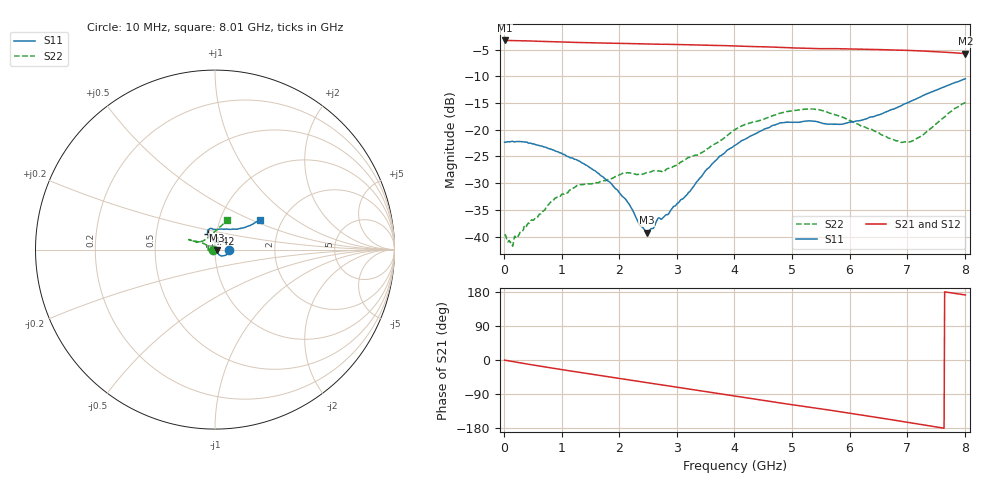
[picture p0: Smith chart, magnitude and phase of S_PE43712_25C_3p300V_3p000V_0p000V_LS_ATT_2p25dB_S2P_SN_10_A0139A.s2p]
! DEVICE ID: PE43712
! File Path: z:\PE43713\PE43713_CHAR_NOM_04292014\AMB\3p300\LS_ATT_2p25dB\PE43713_AMB_3p300V_3p000V_0p000V_LS_ATT_2p25dB_S2P_SN_10_A0139A.s2p
! Serial: 10
! Lot: A0139A
! Temp: 25C
! VDD: 3.300
! VSS: 0.000
! Control_Hi: 3.000
! Control_Lo: 0.000
! Attenuation Step: 2.25dB
! Port 1: RF1
! Port 2: RF2
! ThroughPath:1-2
! IDD: 0.0001467323
! ISS: -1.32e-007
#  Hz  S  RI  R  50
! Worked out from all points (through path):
!   801 points, 10 MHz to 8.01 GHz, reference 50 ohm
!   highest |S21| = -3.29 dB at 10 MHz (marker M1); lowest = -5.7 dB at 8.01 GHz (marker M2)
!   group delay of S21, straight-line fit = 64.5 ps
!   lowest |S11| = -39.3 dB at 2.48 GHz (marker M3), VSWR 1.02, Z = 51.1 - j0.227 ohm
!   |S11| at or under -10 dB: start of sweep to end of sweep
!   |S22| runs from -41.8 to -14.9 dB; largest |S21 - S12| = 0.002
!   S11 on the Smith chart (normalised r, x): 10 MHz: 1.17, -0.00; 4.42 GHz: 0.91, +0.16; 8.01 GHz: 1.55, +0.56
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1e7  0.0765 -0.000436  0.685 -0.00397  0.6847 -0.00374  -0.0103 -0.000149
1.3e8  0.0777 -0.00596  0.6821 -0.0422  0.682 -0.0421  -0.00858 -0.00171
9e8  0.0534 -0.0332  0.6128 -0.2592  0.6127 -0.259  -0.0179 -0.0144
1.35e9  0.0346 -0.0348  0.546 -0.3613  0.5458 -0.3612  -0.0268 -0.015
1.86e9  0.0196 -0.0246  0.4541 -0.4587  0.4541 -0.4586  -0.0342 -0.00646
2.14e9  0.0122 -0.0173  0.3965 -0.504  0.3965 -0.5037  -0.0396 -0.00107
2.35e9  0.0103 -0.00777  0.3501 -0.5332  0.3501 -0.5331  -0.0381 0.00486
2.48e9  0.0106 -0.00222  0.3202 -0.5487  0.3202 -0.5487  -0.0381 0.0113
2.58e9  0.0113 0.00372  0.2969 -0.5586  0.297 -0.5588  -0.0375 0.017
2.68e9  0.0119 0.00899  0.2748 -0.5687  0.275 -0.5686  -0.0347 0.0223
2.86e9  0.0082 0.0142  0.2317 -0.5861  0.2317 -0.5864  -0.0384 0.0204
3.39e9  -0.00427 0.0346  0.0988 -0.6129  0.0988 -0.613  -0.0522 0.0286
3.72e9  -0.012 0.0535  0.0165 -0.6144  0.0165 -0.6143  -0.0681 0.0359
4.01e9  -0.0239 0.0675  -0.0566 -0.6064  -0.0562 -0.6063  -0.0904 0.0434
4.42e9  -0.0406 0.0861  -0.1521 -0.5787  -0.1516 -0.5791  -0.1118 0.0472
4.8e9  -0.0392 0.1092  -0.2352 -0.5413  -0.2347 -0.5415  -0.1337 0.0516
5.35e9  -0.024 0.1183  -0.3364 -0.4688  -0.3363 -0.4684  -0.1468 0.0554
5.86e9  0.011 0.112  -0.4204 -0.3899  -0.4194 -0.3899  -0.1227 0.0472
6.68e9  0.0991 0.1134  -0.5127 -0.2227  -0.5125 -0.2224  -0.0687 0.0471
6.9e9  0.124 0.114  -0.5277 -0.1728  -0.5274 -0.1727  -0.0505 0.0572
7.1e9  0.146 0.1192  -0.5364 -0.126  -0.5357 -0.126  -0.0312 0.0726
8.01e9  0.2506 0.1642  -0.5112 0.0751  -0.5097 0.0742  0.0676 0.1665
